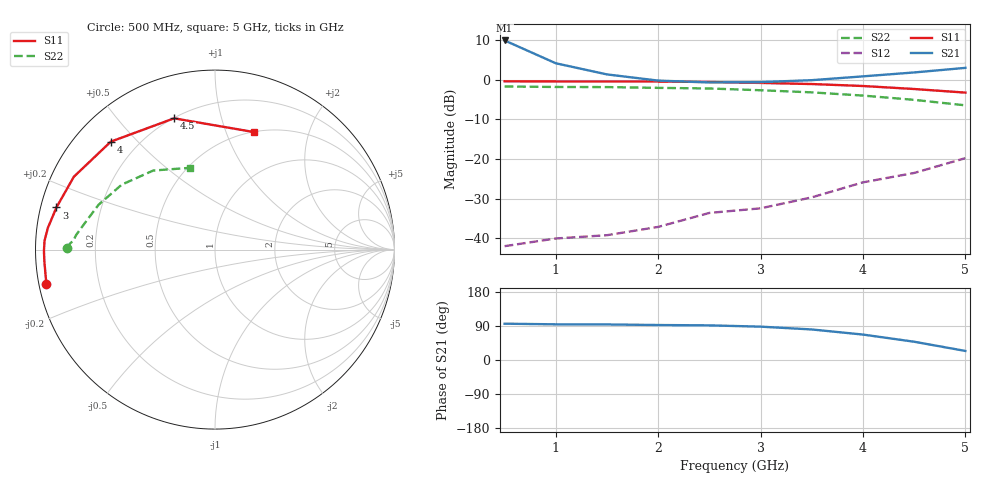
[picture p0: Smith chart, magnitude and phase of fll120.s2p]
# MHZ S MA R 50
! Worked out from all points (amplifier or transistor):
!   10 points, 500 MHz to 5 GHz, reference 50 ohm
!   highest |S21| = 9.9 dB at 500 MHz (marker M1)
!   |S21| within 3 dB of that: start of sweep to 760.7 MHz
!   unconditionally stable (mu >= 1): 637 MHz to end of sweep
!   at 1 GHz: K = 1.54, MAG = 17.8 dB, |S12| = -40.0 dB
!   at 3 GHz: K = 2.27, MAG = 9.6 dB, |S12| = -32.4 dB
!   at 5 GHz: K = 1.49, MAG = 7.3 dB, |S12| = -19.7 dB
!   S11 on the Smith chart (normalised r, x): 500 MHz: 0.02, -0.10; 3 GHz: 0.05, +0.13; 4 GHz: 0.11, +0.42; 4.5 GHz: 0.20, +0.72; 5 GHz: 0.50, +1.26
500  0.959 -168.4  3.136 95.8  0.008 31.0  0.824 179.4
1000  0.953 -176.0  1.617 94.1  0.01 45.7  0.813 178.8
1500  0.953 -179.6  1.17 93.8  0.011 64.3  0.81 177.7
2000  0.951 177.0  0.978 92.3  0.014 82.4  0.792 176.5
2500  0.939 172.6  0.927 91.4  0.021 89.1  0.778 174.0
3000  0.914 165.1  0.936 88.0  0.024 93.2  0.739 168.3
3500  0.885 152.7  0.99 80.6  0.033 94.6  0.695 158.9
4000  0.836 134.0  1.106 67.1  0.051 88.1  0.633 145.1
4500  0.766 107.3  1.239 48.2  0.067 77.3  0.559 128.0
5000  0.69 71.6  1.415 23.9  0.103 60.5  0.477 107.3
